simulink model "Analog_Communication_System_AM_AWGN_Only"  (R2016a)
settings: Solver=ode3  StartTime=0.0  StopTime=6  FixedStep=1/5000000  RelTol=1e-3
libraries: dsparch4 x8, commsynccomp2 x8, simulink x8, commchan3 x1

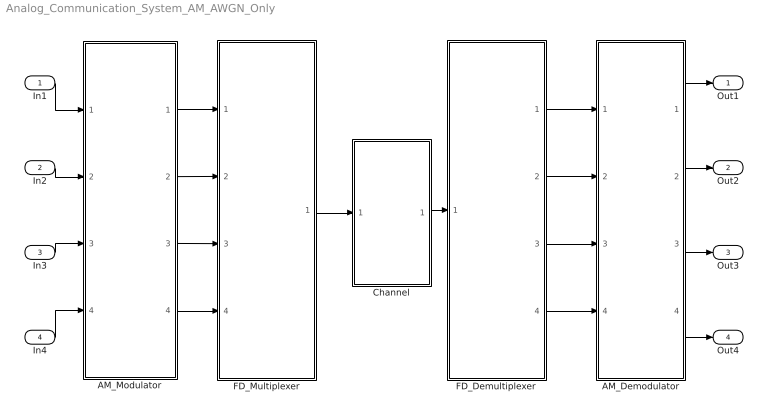
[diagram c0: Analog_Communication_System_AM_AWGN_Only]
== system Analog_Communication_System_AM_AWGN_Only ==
  In1 : Inport
  In2 : Inport  Port=2
  In3 : Inport  Port=3
  In4 : Inport  Port=4
  AM_Demodulator : Subsystem
  AM_Modulator : Subsystem
  Channel : Subsystem
  FD_Demultiplexer : Subsystem
  FD_Multiplexer : Subsystem
  Out1 : Outport
  Out2 : Outport  Port=2
  Out3 : Outport  Port=3
  Out4 : Outport  Port=4
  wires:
  In1/1 -> AM_Modulator/1(In1)
  AM_Modulator/1(Out1) -> FD_Multiplexer/1(In1)
  AM_Modulator/2(Out2) -> FD_Multiplexer/2(In2)
  AM_Modulator/3(Out3) -> FD_Multiplexer/3(In3)
  AM_Modulator/4(Out4) -> FD_Multiplexer/4(In4)
  FD_Multiplexer/1(Out1) -> Channel/1(In1)
  FD_Demultiplexer/2(Out2) -> AM_Demodulator/2(In2)
  FD_Demultiplexer/3(Out3) -> AM_Demodulator/3(In3)
  FD_Demultiplexer/4(Out4) -> AM_Demodulator/4(In4)
  AM_Demodulator/1(Out1) -> Out1/1
  AM_Demodulator/2(Out2) -> Out2/1
  AM_Demodulator/3(Out3) -> Out3/1
  AM_Demodulator/4(Out4) -> Out4/1
  In2/1 -> AM_Modulator/2(In2)
  In3/1 -> AM_Modulator/3(In3)
  In4/1 -> AM_Modulator/4(In4)
  FD_Demultiplexer/1(Out1) -> AM_Demodulator/1(In1)
  Channel/1(Out1) -> FD_Demultiplexer/1(Input)

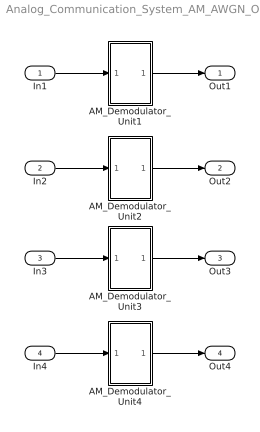
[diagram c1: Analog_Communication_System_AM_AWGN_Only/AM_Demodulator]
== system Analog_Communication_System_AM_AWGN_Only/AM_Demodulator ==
  In1 : Inport
  In2 : Inport  Port=2
  In3 : Inport  Port=3
  In4 : Inport  Port=4
  AM_Demodulator_Unit1 : Subsystem
  AM_Demodulator_Unit2 : Subsystem
  AM_Demodulator_Unit3 : Subsystem
  AM_Demodulator_Unit4 : Subsystem
  Out1 : Outport
  Out2 : Outport  Port=2
  Out3 : Outport  Port=3
  Out4 : Outport  Port=4
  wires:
  In1/1 -> AM_Demodulator_Unit1/1(In1)
  AM_Demodulator_Unit1/1(Out1) -> Out1/1
  In2/1 -> AM_Demodulator_Unit2/1(In1)
  AM_Demodulator_Unit2/1(Out1) -> Out2/1
  In3/1 -> AM_Demodulator_Unit3/1(In1)
  AM_Demodulator_Unit3/1(Out1) -> Out3/1
  In4/1 -> AM_Demodulator_Unit4/1(In1)
  AM_Demodulator_Unit4/1(Out1) -> Out4/1

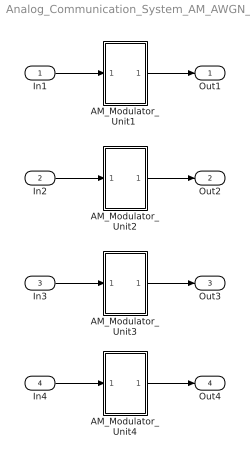
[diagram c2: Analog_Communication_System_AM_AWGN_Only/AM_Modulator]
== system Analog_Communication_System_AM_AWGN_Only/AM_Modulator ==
  In1 : Inport
  In2 : Inport  Port=2
  In3 : Inport  Port=3
  In4 : Inport  Port=4
  "AM_Modulator_Unit1 " : Subsystem
  AM_Modulator_Unit2 : Subsystem
  AM_Modulator_Unit3 : Subsystem
  AM_Modulator_Unit4 : Subsystem
  Out1 : Outport
  Out2 : Outport  Port=2
  Out3 : Outport  Port=3
  Out4 : Outport  Port=4
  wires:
  In1/1 -> "AM_Modulator_Unit1 "/1(In1)
  "AM_Modulator_Unit1 "/1(Out1) -> Out1/1
  AM_Modulator_Unit2/1(Out1) -> Out2/1
  In3/1 -> AM_Modulator_Unit3/1(In1)
  AM_Modulator_Unit3/1(Out1) -> Out3/1
  In4/1 -> AM_Modulator_Unit4/1(In1)
  AM_Modulator_Unit4/1(Out1) -> Out4/1
  In2/1 -> AM_Modulator_Unit2/1(In1)

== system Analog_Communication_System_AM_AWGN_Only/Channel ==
  In1 : Inport
  AWGN Channel : commchan3/AWGN Channel  InputProcessing=Columns as channels (frame based)  seed=67  noiseMode="Signal to noise ratio  (Eb/No)"  EbNodB=20  EsNodB=10  SNRdB=10  bitsPerSym=2  Ps=1  Tsym=1/5000000  variance=1
  Reshape1 : Reshape
  Out1 : Outport
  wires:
  Reshape1/1 -> Out1/1
  In1/1 -> AWGN Channel/1
  AWGN Channel/1 -> Reshape1/1

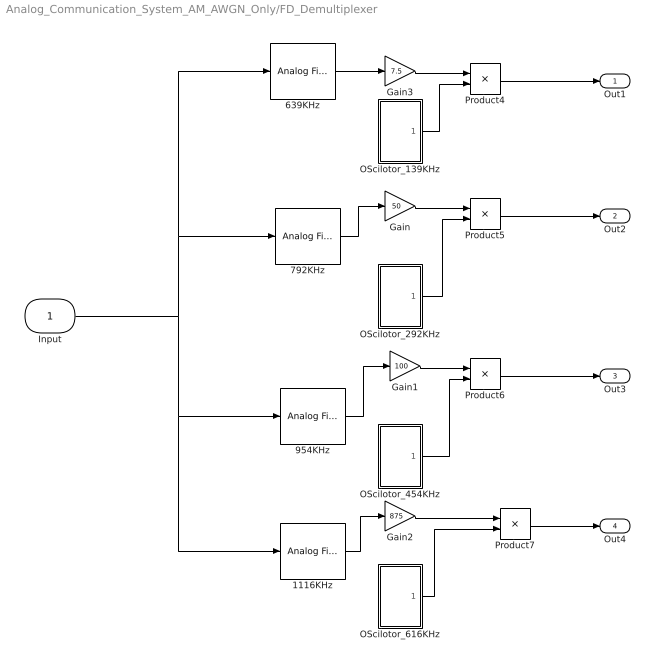
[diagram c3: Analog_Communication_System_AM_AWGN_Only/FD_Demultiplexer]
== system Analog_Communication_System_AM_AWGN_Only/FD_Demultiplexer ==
  Input : Inport
  1116KHz : dsparch4/Analog Filter Design  method=Butterworth  filttype=Bandpass  N=8  Wlo=1066000*2*pi  Whi=1166000*2*pi  Rp=2  Rs=60
  639KHz : dsparch4/Analog Filter Design  method=Butterworth  filttype=Bandpass  N=8  Wlo=589000*2*pi  Whi=689000*2*pi  Rp=2  Rs=40
  792KHz : dsparch4/Analog Filter Design  method=Butterworth  filttype=Bandpass  N=8  Wlo=742000*2*pi  Whi=842000*2*pi  Rp=2  Rs=40
  954KHz : dsparch4/Analog Filter Design  method=Butterworth  filttype=Bandpass  N=8  Wlo=904000*2*pi  Whi=1004000*2*pi  Rp=2  Rs=40
  Gain : Gain  Gain=50
  Gain1 : Gain  Gain=100
  Gain2 : Gain  Gain=875
  Gain3 : Gain  Gain=7.5
  OScilotor_139KHz : Subsystem
  OScilotor_292KHz : Subsystem
  OScilotor_454KHz : Subsystem
  OScilotor_616KHz : Subsystem
  Product{4..7} (4 alike) : Product
  Out1 : Outport
  Out2 : Outport  Port=2
  Out3 : Outport  Port=3
  Out4 : Outport  Port=4
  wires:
  Input/1 -> 1116KHz/1, 954KHz/1, 792KHz/1, 639KHz/1
  OScilotor_139KHz/1(Output) -> Product4/2
  OScilotor_292KHz/1(Output) -> Product5/2
  OScilotor_616KHz/1(Output) -> Product7/2
  OScilotor_454KHz/1(Output) -> Product6/2
  Product5/1 -> Out2/1
  Product4/1 -> Out1/1
  Product6/1 -> Out3/1
  Product7/1 -> Out4/1
  Gain/1 -> Product5/1
  792KHz/1 -> Gain/1
  Gain1/1 -> Product6/1
  954KHz/1 -> Gain1/1
  Gain2/1 -> Product7/1
  1116KHz/1 -> Gain2/1
  639KHz/1 -> Gain3/1
  Gain3/1 -> Product4/1

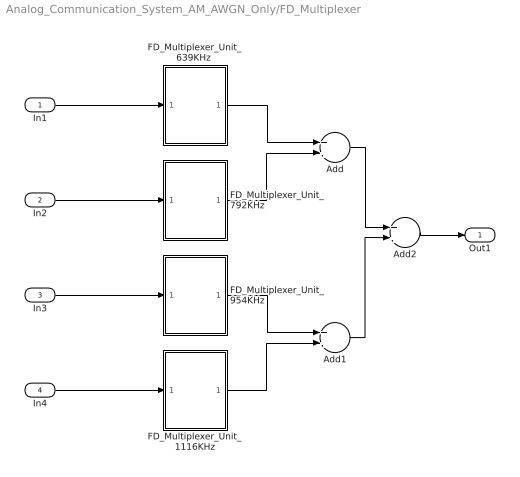
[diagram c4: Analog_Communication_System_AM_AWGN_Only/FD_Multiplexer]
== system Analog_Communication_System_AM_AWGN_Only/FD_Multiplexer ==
  In1 : Inport
  In2 : Inport  Port=2
  In3 : Inport  Port=3
  In4 : Inport  Port=4
  Add : Sum
  Add1 : Sum
  Add2 : Sum
  FD_Multiplexer_Unit_1116KHz : Subsystem
  "FD_Multiplexer_Unit_639KHz " : Subsystem
  FD_Multiplexer_Unit_792KHz : Subsystem
  FD_Multiplexer_Unit_954KHz : Subsystem
  Out1 : Outport
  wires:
  Add2/1 -> Out1/1
  FD_Multiplexer_Unit_792KHz/1(Output) -> Add/2
  FD_Multiplexer_Unit_954KHz/1(Output) -> Add1/1
  FD_Multiplexer_Unit_1116KHz/1(Output) -> Add1/2
  "FD_Multiplexer_Unit_639KHz "/1(Output) -> Add/1
  Add/1 -> Add2/1
  Add1/1 -> Add2/2
  In3/1 -> FD_Multiplexer_Unit_954KHz/1(Input)
  In1/1 -> "FD_Multiplexer_Unit_639KHz "/1(Input)
  In2/1 -> FD_Multiplexer_Unit_792KHz/1(Input)
  In4/1 -> FD_Multiplexer_Unit_1116KHz/1(Input)

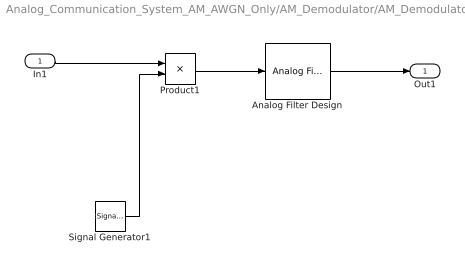
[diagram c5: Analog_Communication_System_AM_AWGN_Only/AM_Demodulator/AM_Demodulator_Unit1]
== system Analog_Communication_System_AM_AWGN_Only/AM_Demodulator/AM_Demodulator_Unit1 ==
  In1 : Inport
  Analog Filter Design : dsparch4/Analog Filter Design  method=Butterworth  filttype=Lowpass  N=8  Wlo=45000*2*pi  Whi=80  Rp=2  Rs=40
  Product1 : Product
  Signal Generator1 : SignalGenerator  Frequency=500000
  Out1 : Outport
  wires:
  Product1/1 -> Analog Filter Design/1
  In1/1 -> Product1/1
  Signal Generator1/1 -> Product1/2
  Analog Filter Design/1 -> Out1/1

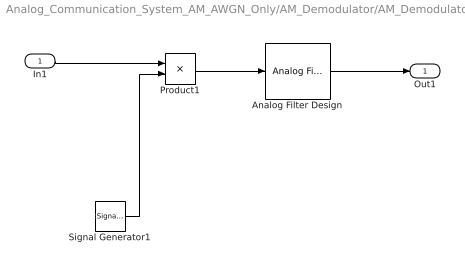
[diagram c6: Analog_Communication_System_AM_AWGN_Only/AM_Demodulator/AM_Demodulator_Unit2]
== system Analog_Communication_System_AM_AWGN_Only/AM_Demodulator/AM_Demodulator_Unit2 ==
  In1 : Inport
  Analog Filter Design : dsparch4/Analog Filter Design  method=Butterworth  filttype=Lowpass  N=8  Wlo=45000*2*pi  Whi=80  Rp=2  Rs=40
  Product1 : Product
  Signal Generator1 : SignalGenerator  Frequency=500000
  Out1 : Outport
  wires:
  Product1/1 -> Analog Filter Design/1
  In1/1 -> Product1/1
  Signal Generator1/1 -> Product1/2
  Analog Filter Design/1 -> Out1/1

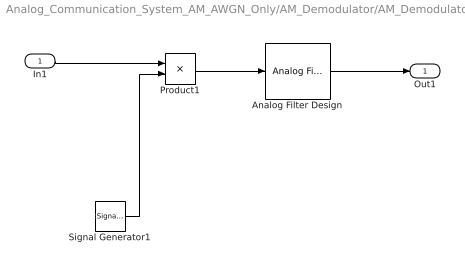
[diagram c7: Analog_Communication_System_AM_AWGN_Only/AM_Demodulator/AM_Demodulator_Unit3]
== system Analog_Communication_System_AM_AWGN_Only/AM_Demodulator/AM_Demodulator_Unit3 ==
  In1 : Inport
  Analog Filter Design : dsparch4/Analog Filter Design  method=Butterworth  filttype=Lowpass  N=8  Wlo=45000*2*pi  Whi=80  Rp=2  Rs=40
  Product1 : Product
  Signal Generator1 : SignalGenerator  Frequency=500000
  Out1 : Outport
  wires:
  Product1/1 -> Analog Filter Design/1
  In1/1 -> Product1/1
  Signal Generator1/1 -> Product1/2
  Analog Filter Design/1 -> Out1/1

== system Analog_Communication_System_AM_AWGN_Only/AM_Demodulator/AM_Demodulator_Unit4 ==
  In1 : Inport
  Analog Filter Design : dsparch4/Analog Filter Design  method=Butterworth  filttype=Lowpass  N=8  Wlo=45000*2*pi  Whi=80  Rp=2  Rs=40
  Product1 : Product
  Signal Generator1 : SignalGenerator  Frequency=500000
  Out1 : Outport
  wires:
  Product1/1 -> Analog Filter Design/1
  In1/1 -> Product1/1
  Signal Generator1/1 -> Product1/2
  Analog Filter Design/1 -> Out1/1

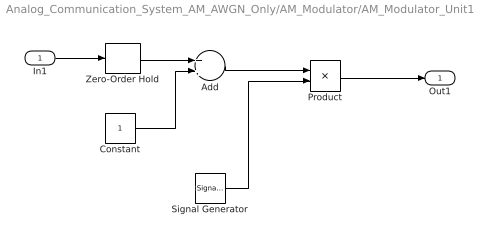
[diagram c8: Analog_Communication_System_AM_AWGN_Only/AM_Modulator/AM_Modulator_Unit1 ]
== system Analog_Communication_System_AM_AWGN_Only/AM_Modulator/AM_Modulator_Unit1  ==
  In1 : Inport
  Add : Sum
  Constant : Constant
  Product : Product
  Signal Generator : SignalGenerator  Frequency=500000
  Zero-Order Hold : ZeroOrderHold  SampleTime=0.0000002
  Out1 : Outport
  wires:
  Constant/1 -> Add/2
  Zero-Order Hold/1 -> Add/1
  Signal Generator/1 -> Product/2
  Product/1 -> Out1/1
  Add/1 -> Product/1
  In1/1 -> Zero-Order Hold/1

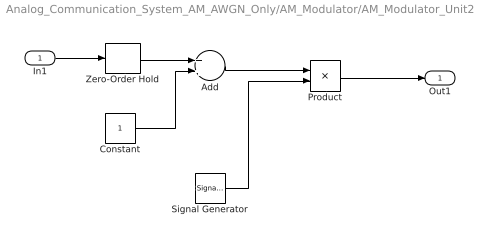
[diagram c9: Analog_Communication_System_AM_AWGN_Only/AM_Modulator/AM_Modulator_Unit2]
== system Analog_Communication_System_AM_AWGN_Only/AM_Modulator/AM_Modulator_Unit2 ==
  In1 : Inport
  Add : Sum
  Constant : Constant
  Product : Product
  Signal Generator : SignalGenerator  Frequency=500000
  Zero-Order Hold : ZeroOrderHold  SampleTime=0.0000002
  Out1 : Outport
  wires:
  Constant/1 -> Add/2
  Zero-Order Hold/1 -> Add/1
  Signal Generator/1 -> Product/2
  Product/1 -> Out1/1
  Add/1 -> Product/1
  In1/1 -> Zero-Order Hold/1

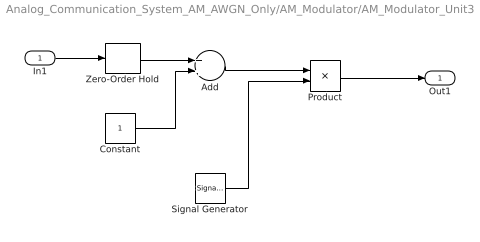
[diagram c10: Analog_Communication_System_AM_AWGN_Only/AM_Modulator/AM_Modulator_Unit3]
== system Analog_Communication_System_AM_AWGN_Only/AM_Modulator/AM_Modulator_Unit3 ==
  In1 : Inport
  Add : Sum
  Constant : Constant
  Product : Product
  Signal Generator : SignalGenerator  Frequency=500000
  Zero-Order Hold : ZeroOrderHold  SampleTime=0.0000002
  Out1 : Outport
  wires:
  Constant/1 -> Add/2
  Zero-Order Hold/1 -> Add/1
  Signal Generator/1 -> Product/2
  Product/1 -> Out1/1
  Add/1 -> Product/1
  In1/1 -> Zero-Order Hold/1

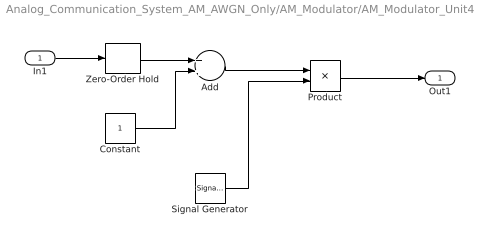
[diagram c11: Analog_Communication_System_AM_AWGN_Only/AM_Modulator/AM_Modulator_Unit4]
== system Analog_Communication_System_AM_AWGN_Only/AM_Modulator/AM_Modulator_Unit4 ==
  In1 : Inport
  Add : Sum
  Constant : Constant
  Product : Product
  Signal Generator : SignalGenerator  Frequency=500000
  Zero-Order Hold : ZeroOrderHold  SampleTime=0.0000002
  Out1 : Outport
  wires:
  Constant/1 -> Add/2
  Zero-Order Hold/1 -> Add/1
  Signal Generator/1 -> Product/2
  Product/1 -> Out1/1
  Add/1 -> Product/1
  In1/1 -> Zero-Order Hold/1

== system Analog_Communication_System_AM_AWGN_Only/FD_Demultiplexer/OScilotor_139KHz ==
  Constant : Constant
  Discrete-Time VCO : commsynccomp2/Discrete-Time VCO  Ac=1  Fc=0  Kc=1000  Ph=0  ts=1/5000000
  Slider Gain : simulink/Math Operations/Slider Gain  low=139  gain=139  high=2070
  Output : Outport
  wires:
  Constant/1 -> Slider Gain/1
  Slider Gain/1 -> Discrete-Time VCO/1
  Discrete-Time VCO/1 -> Output/1

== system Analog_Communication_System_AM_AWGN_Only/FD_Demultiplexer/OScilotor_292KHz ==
  Constant : Constant
  Discrete-Time VCO : commsynccomp2/Discrete-Time VCO  Ac=1  Fc=0  Kc=1000  Ph=0  ts=1/5000000
  Slider Gain : simulink/Math Operations/Slider Gain  low=292  gain=292  high=2070
  Output : Outport
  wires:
  Constant/1 -> Slider Gain/1
  Slider Gain/1 -> Discrete-Time VCO/1
  Discrete-Time VCO/1 -> Output/1

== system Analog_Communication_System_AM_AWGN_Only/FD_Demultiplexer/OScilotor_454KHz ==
  Constant : Constant
  Discrete-Time VCO : commsynccomp2/Discrete-Time VCO  Ac=1  Fc=0  Kc=1000  Ph=0  ts=1/5000000
  Slider Gain : simulink/Math Operations/Slider Gain  low=454  gain=454  high=2070
  Output : Outport
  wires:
  Constant/1 -> Slider Gain/1
  Slider Gain/1 -> Discrete-Time VCO/1
  Discrete-Time VCO/1 -> Output/1

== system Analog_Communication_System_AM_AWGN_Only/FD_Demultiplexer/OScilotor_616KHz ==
  Constant : Constant
  Discrete-Time VCO : commsynccomp2/Discrete-Time VCO  Ac=1  Fc=0  Kc=1000  Ph=0  ts=1/5000000
  Slider Gain : simulink/Math Operations/Slider Gain  low=616  gain=616  high=2070
  Output : Outport
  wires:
  Constant/1 -> Slider Gain/1
  Slider Gain/1 -> Discrete-Time VCO/1
  Discrete-Time VCO/1 -> Output/1

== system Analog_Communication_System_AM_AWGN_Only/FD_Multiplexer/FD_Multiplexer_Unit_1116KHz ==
  Input : Inport
  Carrier Generator : Subsystem
  Product : Product
  Output : Outport
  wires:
  Input/1 -> Product/1
  Product/1 -> Output/1
  Carrier Generator/1(Carrier) -> Product/2

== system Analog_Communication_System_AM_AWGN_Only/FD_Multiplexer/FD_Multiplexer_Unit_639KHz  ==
  Input : Inport
  Carrier Generator : Subsystem
  Product : Product
  Output : Outport
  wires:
  Product/1 -> Output/1
  Input/1 -> Product/1
  Carrier Generator/1(Carrier) -> Product/2

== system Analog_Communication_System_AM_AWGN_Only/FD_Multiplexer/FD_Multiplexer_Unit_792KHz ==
  Input : Inport
  Carrier Generator : Subsystem
  Product : Product
  Output : Outport
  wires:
  Product/1 -> Output/1
  Input/1 -> Product/1
  Carrier Generator/1(Carrier) -> Product/2

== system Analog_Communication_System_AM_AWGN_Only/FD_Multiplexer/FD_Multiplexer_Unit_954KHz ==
  Input : Inport
  Carrier Generator : Subsystem
  Product : Product
  Output : Outport
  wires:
  Input/1 -> Product/1
  Product/1 -> Output/1
  Carrier Generator/1(Carrier) -> Product/2

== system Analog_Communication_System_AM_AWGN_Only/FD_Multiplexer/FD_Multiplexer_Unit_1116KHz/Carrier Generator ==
  Constant1 : Constant
  Discrete-Time VCO : commsynccomp2/Discrete-Time VCO  Ac=1  Fc=0  Kc=1000  Ph=0  ts=1/5000000
  Slider Gain : simulink/Math Operations/Slider Gain  low=550  gain=616  high=2500
  Carrier : Outport
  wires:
  Discrete-Time VCO/1 -> Carrier/1
  Slider Gain/1 -> Discrete-Time VCO/1
  Constant1/1 -> Slider Gain/1

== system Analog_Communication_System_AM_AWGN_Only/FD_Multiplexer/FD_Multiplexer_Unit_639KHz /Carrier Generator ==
  Constant1 : Constant
  Discrete-Time VCO : commsynccomp2/Discrete-Time VCO  Ac=1  Fc=0  Kc=1000  Ph=0  ts=1/5000000
  Slider Gain : simulink/Math Operations/Slider Gain  low=0  gain=139  high=1605
  Carrier : Outport
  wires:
  Discrete-Time VCO/1 -> Carrier/1
  Slider Gain/1 -> Discrete-Time VCO/1
  Constant1/1 -> Slider Gain/1

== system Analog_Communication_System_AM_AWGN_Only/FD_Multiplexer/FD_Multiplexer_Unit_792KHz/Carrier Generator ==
  Constant1 : Constant
  Discrete-Time VCO : commsynccomp2/Discrete-Time VCO  Ac=1  Fc=0  Kc=1000  Ph=0  ts=1/5000000
  Slider Gain : simulink/Math Operations/Slider Gain  low=292  gain=292  high=1605
  Carrier : Outport
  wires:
  Discrete-Time VCO/1 -> Carrier/1
  Slider Gain/1 -> Discrete-Time VCO/1
  Constant1/1 -> Slider Gain/1

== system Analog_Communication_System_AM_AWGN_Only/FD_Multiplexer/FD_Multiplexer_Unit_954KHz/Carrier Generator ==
  Constant1 : Constant
  Discrete-Time VCO : commsynccomp2/Discrete-Time VCO  Ac=1  Fc=0  Kc=1000  Ph=0  ts=1/5000000
  Slider Gain : simulink/Math Operations/Slider Gain  low=454  gain=454  high=1605
  Carrier : Outport
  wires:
  Discrete-Time VCO/1 -> Carrier/1
  Slider Gain/1 -> Discrete-Time VCO/1
  Constant1/1 -> Slider Gain/1
